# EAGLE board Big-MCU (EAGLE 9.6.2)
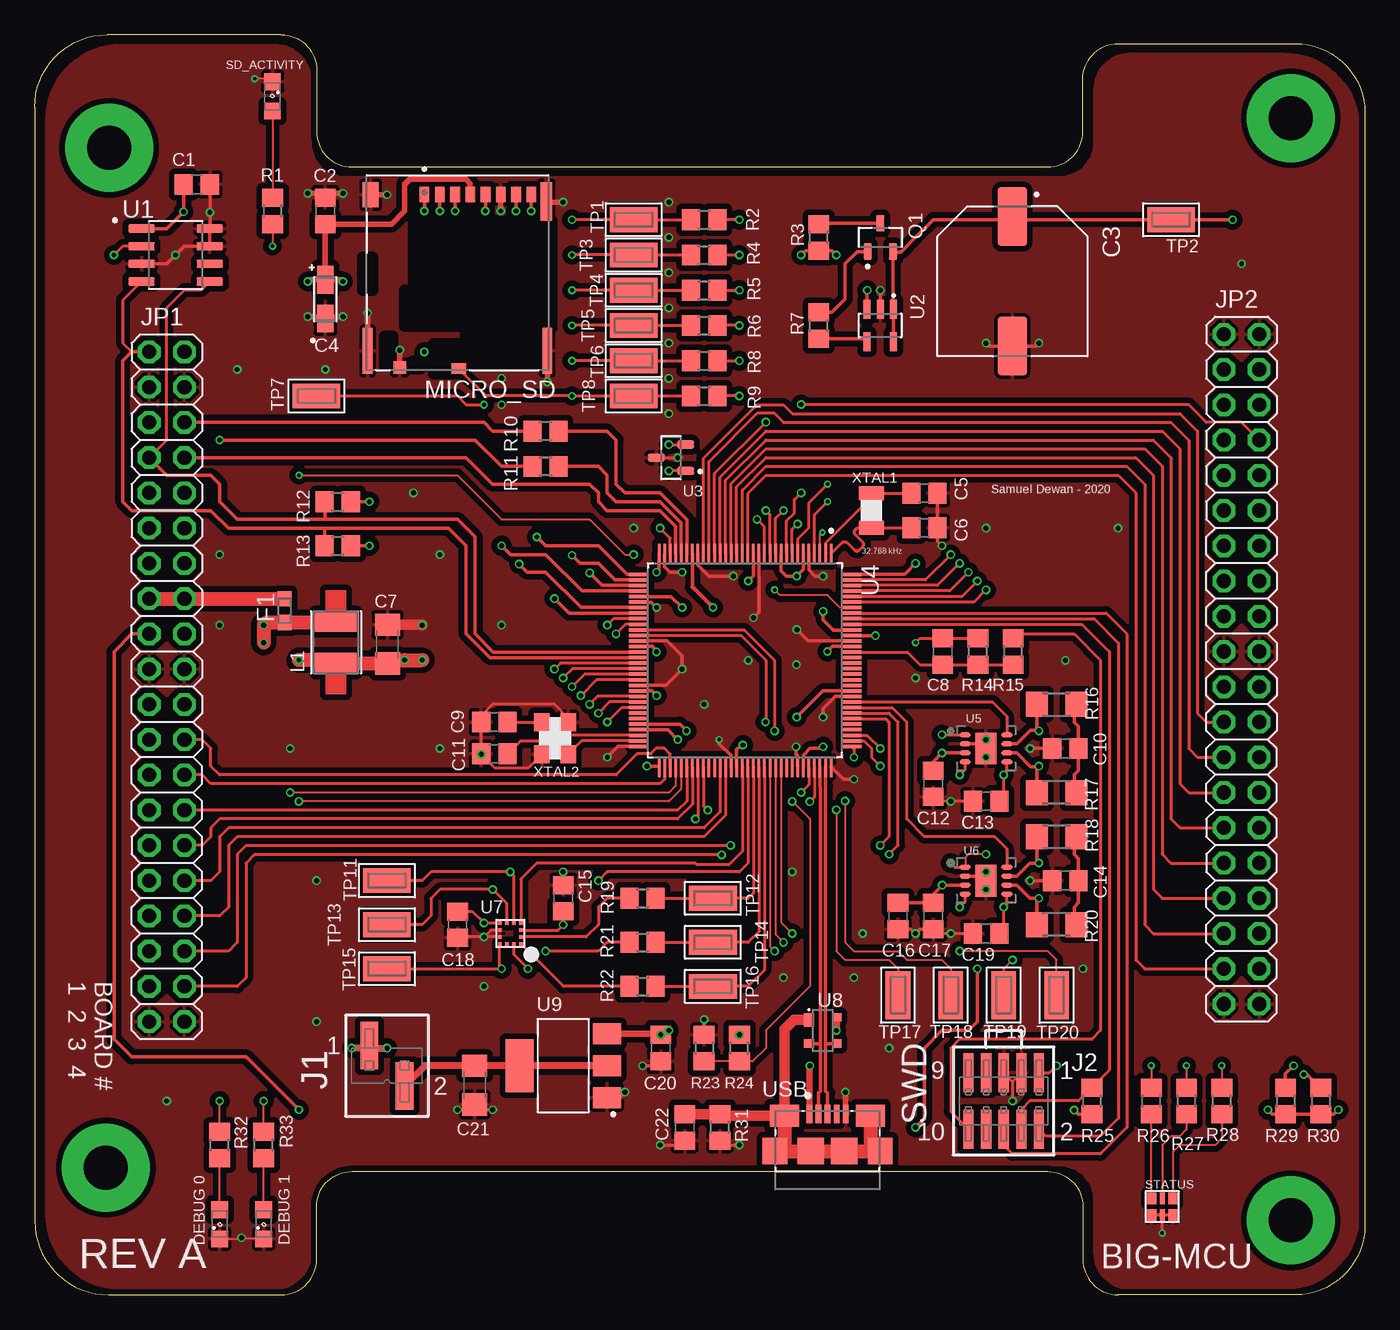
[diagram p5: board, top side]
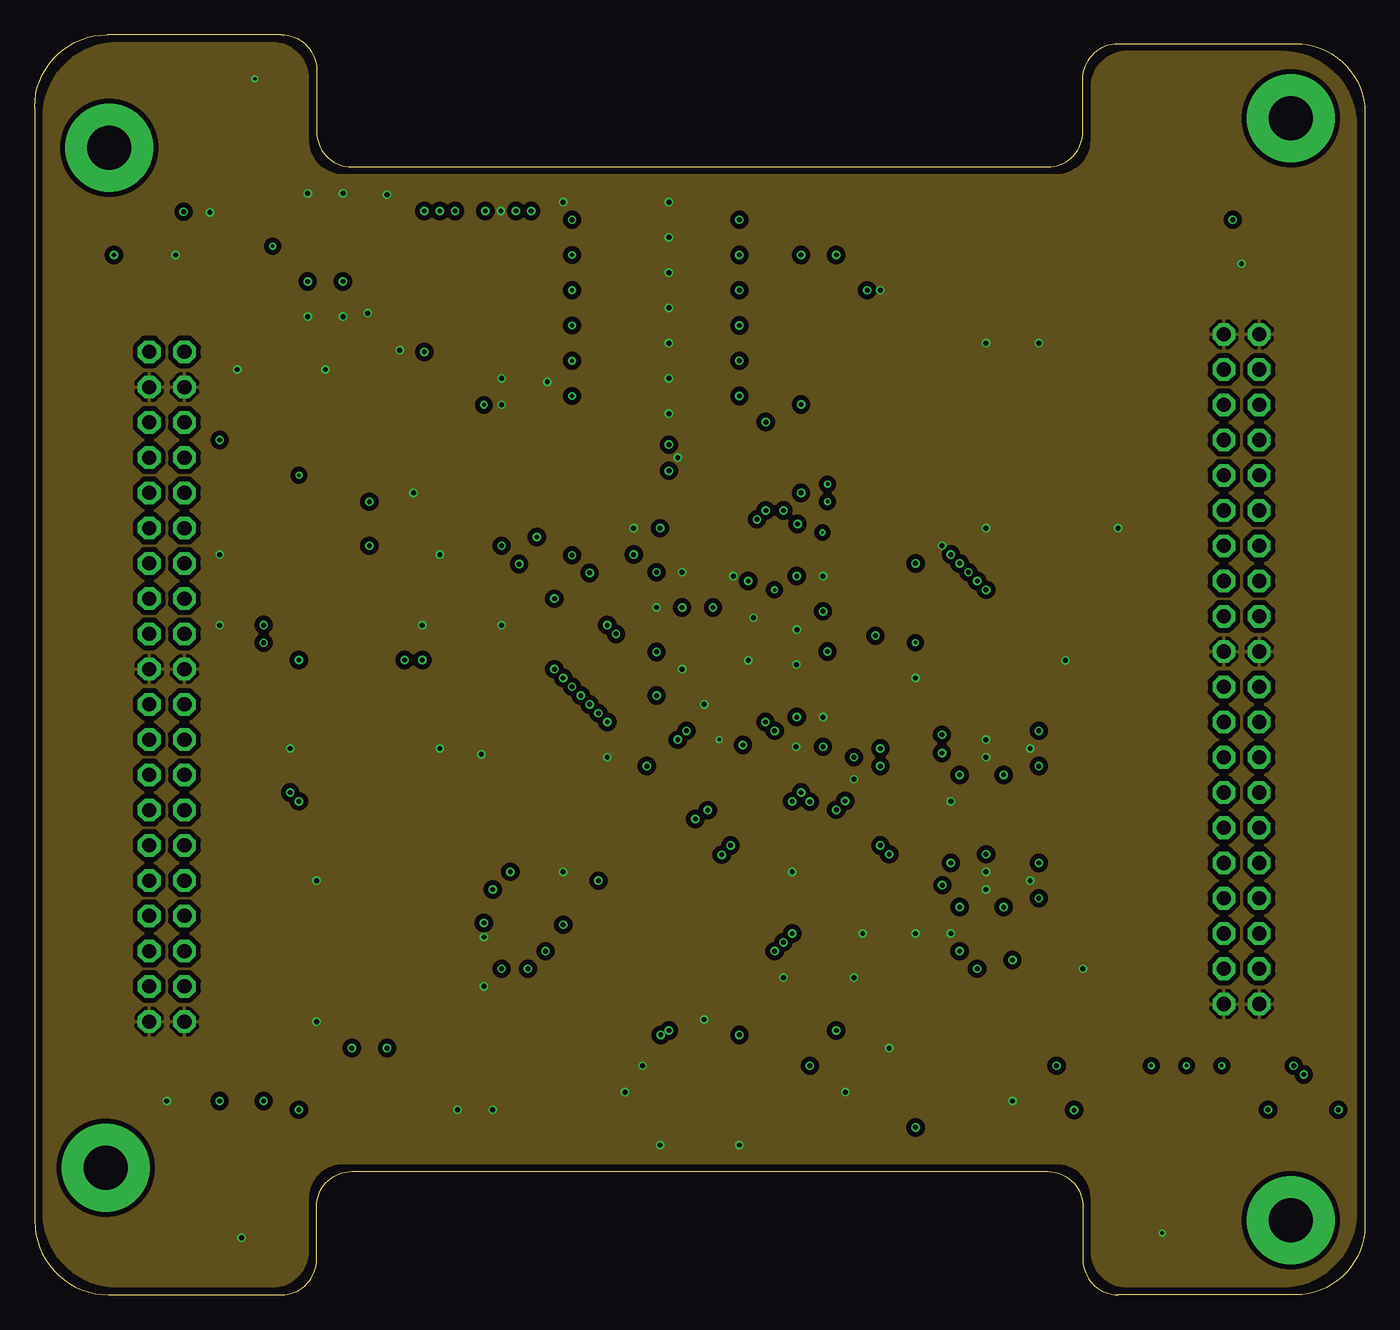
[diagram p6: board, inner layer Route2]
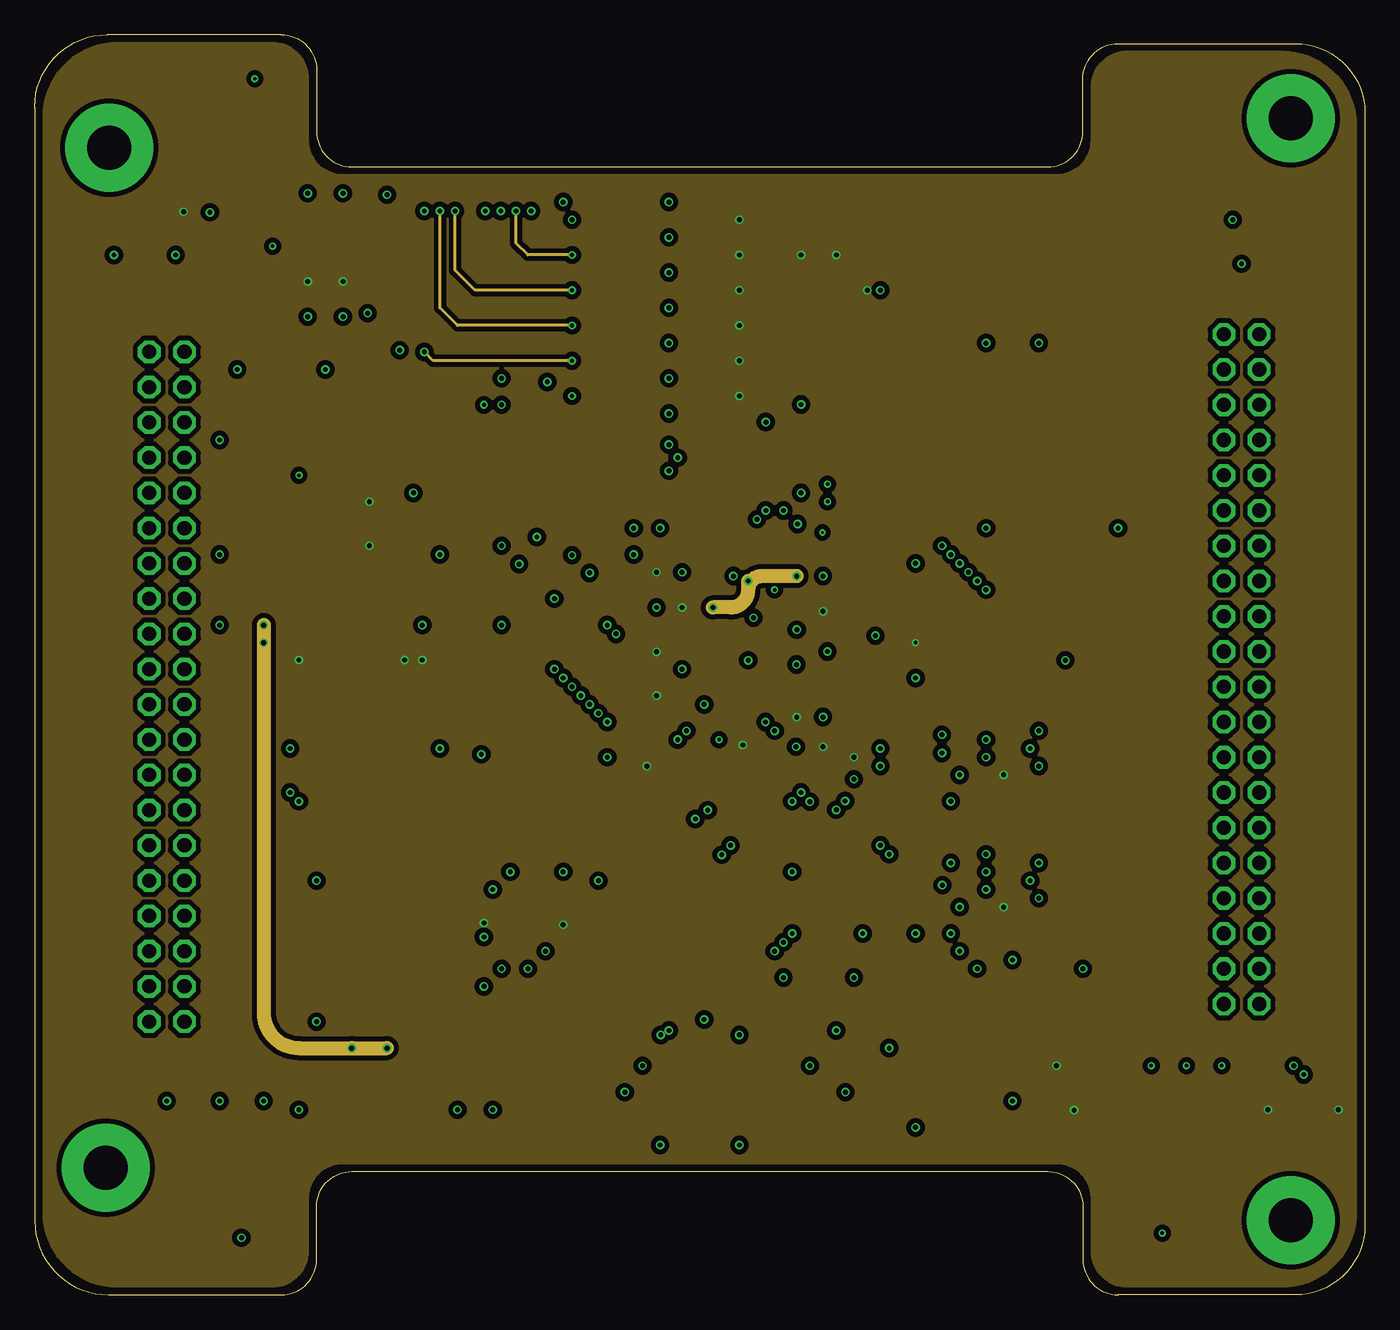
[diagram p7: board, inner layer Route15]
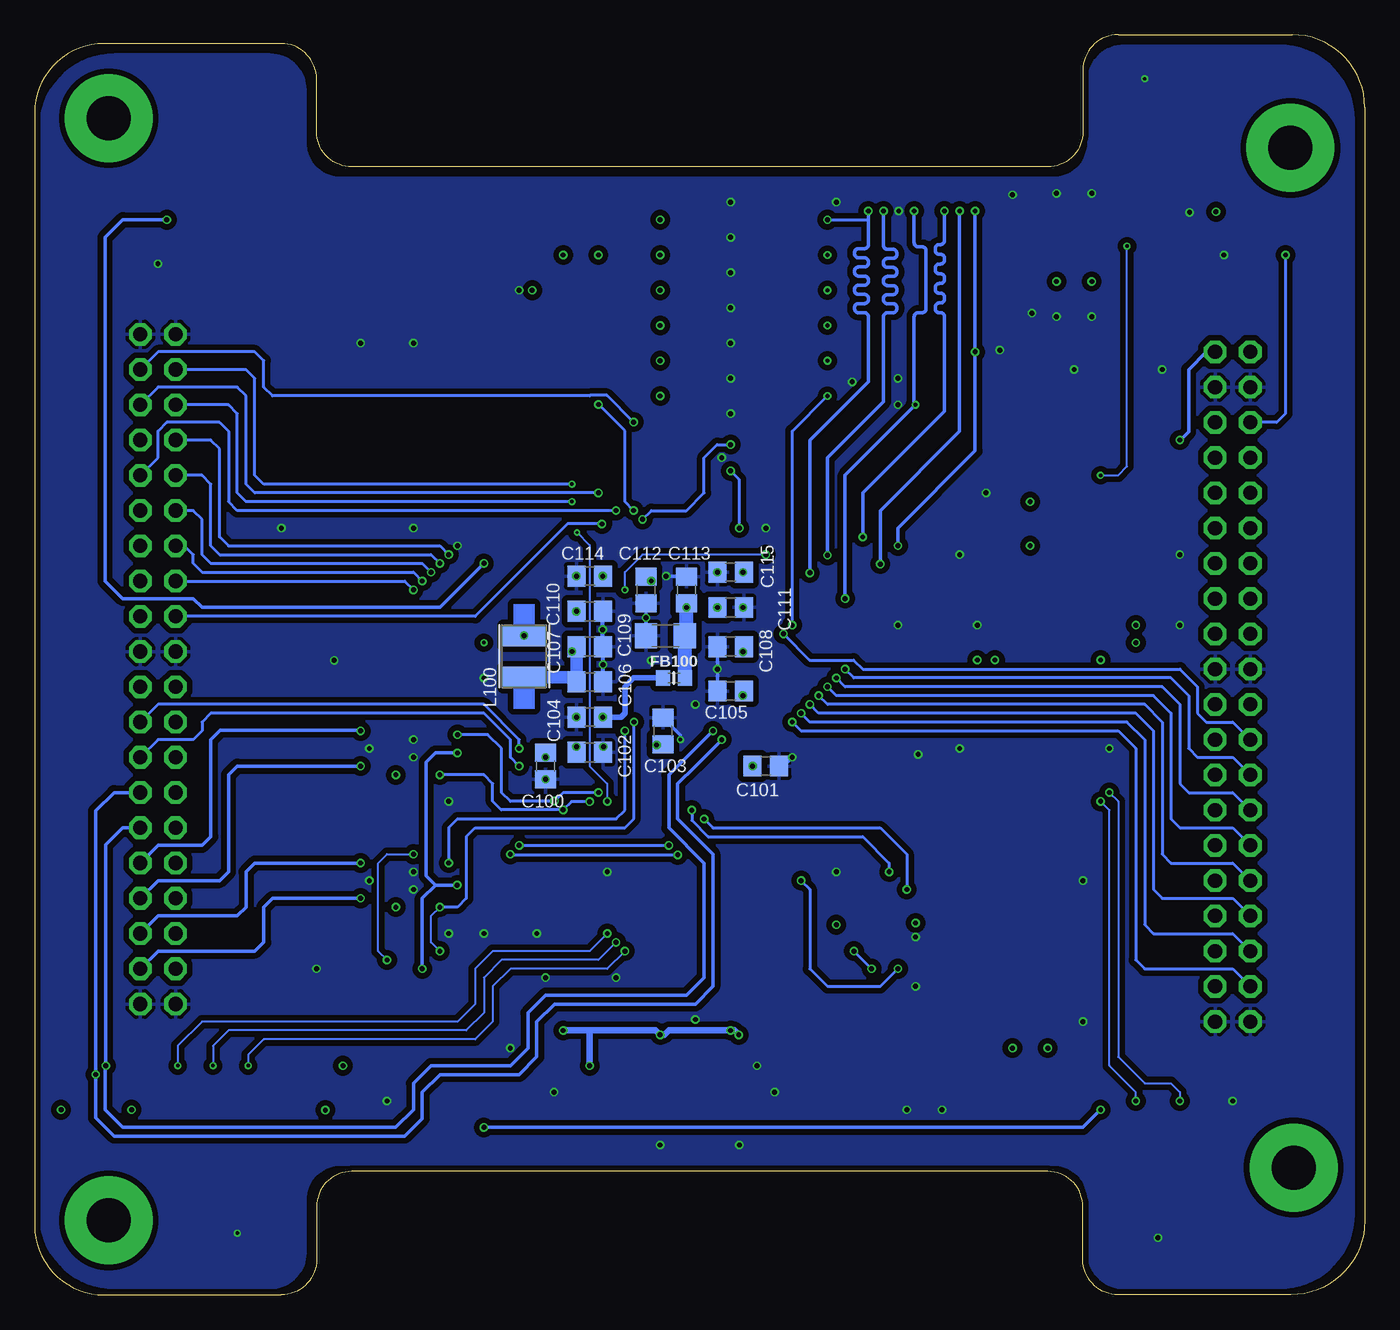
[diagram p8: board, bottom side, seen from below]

Size 95.89 x 90.81 mm. Coordinates in mm from the lower left corner, seen from the top.
Outline: 0,85.57 0,5.33 arc90 5.33,0 17.78,0 arc90 20.32,2.54 20.32,6.35 arc-90 22.86,8.89 73.03,8.89 arc-90 75.56,6.35 75.56,2.54 arc90 78.11,0 90.89,0 arc90 95.89,5 95.89,85.17 arc90 90.89,90.17 78.11,90.17 arc90 75.56,87.63 75.56,83.82 arc-90 73.03,81.28 22.86,81.28 arc-90 20.32,83.82 20.32,88.27 arc90 17.78,90.81 5.23,90.81 arc90 0,85.57
Copper layers (1+2*15+16): Top 0.035mm / dielectric 0.2mm / Route2 0.0175mm / dielectric 1.065mm / Route15 0.0175mm / dielectric 0.2mm / Bottom 0.035mm
Design rules "JLC 4 Layer *": minimum track width 5mil, minimum drill 0.2mm, track to track 3.5mil, track to pad 3.5mil, pad to pad 5mil, via to via 10mil, smd to smd 0mil, copper to edge 10mil, drill to drill 10mil, minimum pad ring 12mil, minimum via ring 5mil, stop-mask expansion 4mil, vias tented up to drill 0mil, thermal gap 10mil
Net classes: 2 diff pairs: width 0.254 mm

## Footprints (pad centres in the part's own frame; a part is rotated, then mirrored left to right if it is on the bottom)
PC/104-MOUNTING-HOLE = drill 3.175 pad 6.35: GND 0,0
C0805 = smd 1.3 x 1.5: 1 -0.95,0; 2 0.95,0
CAPAE1080X580N = smd 4.24 x 2.13: 1 -4.665,0; 2 4.665,0
1206-POL = smd 2 x 1.2: + 1.4,0; - -1.4,0
C1206 = smd 1.6 x 1.8: 1 -1.4,0; 2 1.4,0
SML0805 = smd 1.2 x 1.2: A 1.05,0; C -1.05,0
FUS0603_TYCO = smd 1.092 x 0.991: 1 -0.851,0; 2 0.851,0
0603 = smd 1 x 1.1: 1 -0.794,0; 2 0.794,0
TSM-102-01-L-SV = smd 1.27 x 3.43: 1 -1.27,1.46; 2 1.27,-1.46
SAMTEC-FTSH-105-01-X-DV = smd 0.74 x 2.79: 1 -2.54,-2.032; 2 -2.54,2.032; 3 -1.27,-2.032; 4 -1.27,2.032; 5 0,-2.032; 6 0,2.032; 7 1.27,-2.032; 8 1.27,2.032; 9 2.54,-2.032; 10 2.54,2.032
2X20 = drill 1.016 octagon: 1 -24.13,-1.27; 2 -24.13,1.27; 3 -21.59,-1.27; 4 -21.59,1.27; 5 -19.05,-1.27; 6 -19.05,1.27; 7 -16.51,-1.27; 8 -16.51,1.27; 9 -13.97,-1.27; 10 -13.97,1.27; 11 -11.43,-1.27; 12 -11.43,1.27; 13 -8.89,-1.27; 14 -8.89,1.27; 15 -6.35,-1.27; 16 -6.35,1.27; 17 -3.81,-1.27; 18 -3.81,1.27; 19 -1.27,-1.27; 20 -1.27,1.27; 21 1.27,-1.27; 22 1.27,1.27; 23 3.81,-1.27; 24 3.81,1.27; 25 6.35,-1.27; 26 6.35,1.27; 27 8.89,-1.27; 28 8.89,1.27; 29 11.43,-1.27; 30 11.43,1.27; 31 13.97,-1.27; 32 13.97,1.27; 33 16.51,-1.27; 34 16.51,1.27; 35 19.05,-1.27; 36 19.05,1.27; 37 21.59,-1.27; 38 21.59,1.27; 39 24.13,-1.27; 40 24.13,1.27
LQH43PN100M26L = smd 1.5 x 3: 1 -1.5,0; 2 1.5,0
MOLEX_503398-1892 = smd 0.7 x 1.1: 1 -3.65,6.895; 2 -2.55,6.895; 3 -1.45,6.895; 4 -0.35,6.895; 5 0.75,6.895; 6 1.85,6.895; 7 2.95,6.895; 8 4.05,6.895 | smd 0.9 x 0.93: 9 -5.44,-5.57 | smd 1.05 x 0.78: 10 -1.175,-5.645 | smd 1.14 x 1.83: P1 -7.53,6.88 | smd 0.86 x 2.8: P2 5.13,6.395 | smd 0.7 x 3.33: P3 -7.75,-4.37; P4 5.21,-4.37
SOT91P240X110-3N = smd 1.18 x 0.61: 1 -1.025,0.915; 2 -1.025,-0.915; 3 1.025,0
R0805 = smd 1.3 x 1.5: 1 -0.95,0; 2 0.95,0
R1206 = smd 1.6 x 1.803: 1 -1.422,0; 2 1.422,0
MSL0402RGB = smd 0.67 x 0.83: P1 0.77,-0.585; P3 -0.77,-0.585; P4 0.77,0.585; P6 -0.77,0.585 | smd 0.37 x 0.83: P2 0,-0.585; P5 0,0.585
KEYSTONE_5015 = smd 3.43 x 1.78: 1 0,0
SOIC8 = smd 1.91 x 0.6: 1 -2.46,1.905; 2 -2.46,0.635; 3 -2.46,-0.635; 4 -2.46,-1.905; 5 2.46,-1.905; 6 2.46,-0.635; 7 2.46,0.635; 8 2.46,1.905
SOT95P285X145-5N = smd 1.37 x 0.59: 1 -1.175,0.95; 2 -1.175,0; 3 -1.175,-0.95; 4 1.175,-0.95; 5 1.175,0.95
SOT95P237X112-3N = smd 1.23 x 0.59: 1 -1.06,0.95; 2 -1.06,-0.95; 3 1.06,0
QFP40P1600X1600X120-128N = smd 1.47 x 0.24: 1 -7.67,6.2; 2 -7.67,5.8; 3 -7.67,5.4; 4 -7.67,5; 5 -7.67,4.6; 6 -7.67,4.2; 7 -7.67,3.8; 8 -7.67,3.4; 9 -7.67,3; 10 -7.67,2.6; 11 -7.67,2.2; 12 -7.67,1.8; 13 -7.67,1.4; 14 -7.67,1; 15 -7.67,0.6; 16 -7.67,0.2; 17 -7.67,-0.2; 18 -7.67,-0.6; 19 -7.67,-1; 20 -7.67,-1.4; 21 -7.67,-1.8; 22 -7.67,-2.2; 23 -7.67,-2.6; 24 -7.67,-3; 25 -7.67,-3.4; 26 -7.67,-3.8; 27 -7.67,-4.2; 28 -7.67,-4.6; 29 -7.67,-5; 30 -7.67,-5.4; 31 -7.67,-5.8; 32 -7.67,-6.2; 65 7.67,-6.2; 66 7.67,-5.8; 67 7.67,-5.4; 68 7.67,-5; 69 7.67,-4.6; 70 7.67,-4.2; 71 7.67,-3.8; 72 7.67,-3.4; 73 7.67,-3; 74 7.67,-2.6; 75 7.67,-2.2; 76 7.67,-1.8; 77 7.67,-1.4; 78 7.67,-1; 79 7.67,-0.6; 80 7.67,-0.2; 81 7.67,0.2; 82 7.67,0.6; 83 7.67,1; 84 7.67,1.4; 85 7.67,1.8; 86 7.67,2.2; 87 7.67,2.6; 88 7.67,3; 89 7.67,3.4; 90 7.67,3.8; 91 7.67,4.2; 92 7.67,4.6; 93 7.67,5; 94 7.67,5.4; 95 7.67,5.8; 96 7.67,6.2 | smd 0.24 x 1.47: 33 -6.2,-7.67; 34 -5.8,-7.67; 35 -5.4,-7.67; 36 -5,-7.67; 37 -4.6,-7.67; 38 -4.2,-7.67; 39 -3.8,-7.67; 40 -3.4,-7.67; 41 -3,-7.67; 42 -2.6,-7.67; 43 -2.2,-7.67; 44 -1.8,-7.67; 45 -1.4,-7.67; 46 -1,-7.67; 47 -0.6,-7.67; 48 -0.2,-7.67; 49 0.2,-7.67; 50 0.6,-7.67; 51 1,-7.67; 52 1.4,-7.67; 53 1.8,-7.67; 54 2.2,-7.67; 55 2.6,-7.67; 56 3,-7.67; 57 3.4,-7.67; 58 3.8,-7.67; 59 4.2,-7.67; 60 4.6,-7.67; 61 5,-7.67; 62 5.4,-7.67; 63 5.8,-7.67; 64 6.2,-7.67; 97 6.2,7.67; 98 5.8,7.67; 99 5.4,7.67; 100 5,7.67; 101 4.6,7.67; 102 4.2,7.67; 103 3.8,7.67; 104 3.4,7.67; 105 3,7.67; 106 2.6,7.67; 107 2.2,7.67; 108 1.8,7.67; 109 1.4,7.67; 110 1,7.67; 111 0.6,7.67; 112 0.2,7.67; 113 -0.2,7.67; 114 -0.6,7.67; 115 -1,7.67; 116 -1.4,7.67; 117 -1.8,7.67; 118 -2.2,7.67; 119 -2.6,7.67; 120 -3,7.67; 121 -3.4,7.67; 122 -3.8,7.67; 123 -4.2,7.67; 124 -4.6,7.67; 125 -5,7.67; 126 -5.4,7.67; 127 -5.8,7.67; 128 -6.2,7.67
VDFN8 = smd 2.3 x 1.5: EP 0,0 | smd 0.35 x 0.8: P1 -0.975,-1.5; P2 -0.325,-1.5; P3 0.325,-1.5; P4 0.975,-1.5; P5 0.975,1.5; P6 0.325,1.5; P7 -0.325,1.5; P8 -0.975,1.5
KX134-1211 = smd 0.275 x 0.25: 1 -0.762,0.75; 2 -0.762,0.25; 3 -0.762,-0.25; 4 -0.762,-0.75; 7 0.762,-0.75; 8 0.762,-0.25; 9 0.762,0.25; 10 0.762,0.75 | smd 0.25 x 0.275: 5 -0.25,-0.762; 6 0.25,-0.762; 11 0.25,0.762; 12 -0.25,0.762
SOT143B = smd 1 x 0.7: 1 -0.75,-1 | smd 0.6 x 0.7: 2 0.95,-1; 3 0.95,1; 4 -0.95,1
SOT223 = smd 1.5 x 2: 1 -2.3,-3.15; 2 0,-3.15; 3 2.3,-3.15 | smd 3.8 x 2: 4 0,3.15
10118192-0001LF = smd 0.4 x 1.35: 1 -1.3,2.54; 2 -0.65,2.54; 3 0,2.54; 4 0.65,2.54; 5 1.3,2.54 | smd 2.1 x 1.6: SH1 -3.1,2.415; SH2 3.1,2.415 | smd 1.8 x 1.9: SH3 -3.8,-0.135; SH6 3.8,-0.135 | smd 1.9 x 1.9: SH4 -1.2,-0.135; SH5 1.2,-0.135
CM7V-T1A-32.768KHZ-12.5PF-10PPM-TA-QC = smd 1 x 1.8: P$1 -1.25,0; P$2 1.25,0
RH100-12.000-12-1010-EXT-TR = smd 1.3 x 1.1: P1 -1.15,-0.95; P2 1.15,-0.95; P3 1.15,0.95; P4 -1.15,0.95

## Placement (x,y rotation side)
$$U$1  PS/104-MOUNTING-HOLE  [PC/104-MOUNTING-HOLE]  5.13,9.17 0 top
C1  0.1 µF  [C0805]  11.68,80.01 0 top
C2  0.1 µF  [C0805]  20.95,78.11 90 top
C3  FC0H473ZFTBR24  [CAPAE1080X580N]  70.48,73.03 270 top
C4  TAJA106K010RNJ  [1206-POL]  20.95,71.75 90 top
C5  22 pF  [C0805]  64.14,57.76 180 top
C6  22 pF  [C0805]  64.14,55.27 180 top
C7  10 µF  [C1206]  25.43,46.89 90 top
C8  100 pF  [C0805]  65.46,46.35 270 top
C9  18 pF  [C0805]  33.15,41.27 0 top
C10  4.7 µF  [C0805]  74.3,39.37 180 top
C11  18 pF  [C0805]  33.15,38.99 0 top
C12  0.1 µF  [C0805]  64.77,36.83 90 top
C13  0.1 µF  [C0805]  68.58,35.56 0 top
C14  4700 pF  [C0805]  74.3,29.84 180 top
C15  0.1µF  [C0805]  38.1,28.57 90 top
C16  4.7 µF  [C0805]  62.23,27.3 90 top
C17  0.1 µF  [C0805]  64.77,27.3 90 top
C18  0.1 µF  [C0805]  30.48,26.67 270 top
C19  0.1 µF  [C0805]  68.58,26.04 0 top
C20  0.1 µF  [C0805]  45.14,17.78 270 top
C21  10 µF  [C1206]  31.72,15.11 270 top
C22  4.7 nF  [C0805]  46.86,12.06 270 top
C100  0.1 µF  [C0805]  59.05,38.1 270 bottom
C101  0.1 µF  [C0805]  43.18,38.1 0 bottom
C102  0.1 µF  [C0805]  55.88,39.09 0 bottom
C103  0.1 µF  [C0805]  50.6,40.64 90 bottom
C104  0.1 µF  [C0805]  55.88,41.63 180 bottom
C105  0.1 µF  [C0805]  45.72,43.51 180 bottom
C106  4.7 µF  [C0805]  55.88,44.17 0 bottom
C107  0.1 µF  [C0805]  55.88,46.71 0 bottom
C108  0.1 µF  [C0805]  45.72,46.71 180 bottom
C109  10 µF  [C1206]  50.42,47.5 180 bottom
C110  0.1 µF  [C0805]  55.88,49.25 0 bottom
C111  0.1 µF  [C0805]  45.72,49.53 0 bottom
C112  0.1 µF  [C0805]  51.82,50.8 270 bottom
C113  0.1 µF  [C0805]  48.9,50.8 90 bottom
C114  0.1 µF  [C0805]  55.88,51.79 180 bottom
C115  0.1 µF  [C0805]  45.72,52.07 180 bottom
DEBUG1  [SML0805]  13.34,5.08 90 top
DEBUG2  [SML0805]  16.51,5.08 90 top
F1  0603SFF150F/32-2  [FUS0603_TYCO]  18.02,49.3 270 top
FB100  BLM18PG471SN1D  [0603]  49.81,44.45 0 bottom
J1  TSM-102-01-L-SVJ  [TSM-102-01-L-SV]  25.4,16.51 0 top
J2  SAMTEC-FTSH-105-01-X-DVJ  [SAMTEC-FTSH-105-01-X-DV]  69.85,13.97 180 top
JP1  [2X20]  9.53,43.81 270 top
JP2  [2X20]  87,45.09 270 top
L1  LQH43PN100M26L  [LQH43PN100M26L]  21.72,47.02 270 top
L100  LQH43PN100M26L  [LQH43PN100M26L]  60.6,46 270 bottom
MICRO_SD  503398-1892  [MOLEX_503398-1892]  31.75,72.39 0 top
Q1  DMG2305UX-13  [SOT91P240X110-3N]  60.96,76.2 90 top
R1  22 kΩ  [R0805]  17.14,78.11 270 top
R2  100 kΩ  [R0805]  48.26,77.47 0 top
R3  220 Ω  [R0805]  56.52,76.2 90 top
R4  100 kΩ  [R0805]  48.26,74.93 0 top
R5  10 kΩ  [R0805]  48.26,72.39 0 top
R6  100 kΩ  [R0805]  48.26,69.85 0 top
R7  1 kΩ  [R0805]  56.52,69.85 90 top
R8  100 kΩ  [R0805]  48.26,67.31 0 top
R9  10 kΩ  [R0805]  48.26,64.77 0 top
R10  33 Ω  [R0805]  36.83,62.23 180 top
R11  33 Ω  [R0805]  36.83,59.69 180 top
R12  2.2 kΩ  [R0805]  21.84,57.15 0 top
R13  2.2 kΩ  [R0805]  21.84,53.98 0 top
R14  2.2 kΩ  [R0805]  68,46.35 90 top
R15  330 Ω  [R0805]  70.54,46.35 90 top
R16  60.4 Ω  [R1206]  73.66,42.55 180 top
R17  60.4 Ω  [R1206]  73.66,36.2 0 top
R18  60.4 Ω  [R1206]  73.66,33.02 180 top
R19  33 Ω  [R0805]  43.81,28.57 0 top
R20  60.4 Ω  [R1206]  73.66,26.67 0 top
R21  33 Ω  [R0805]  43.81,25.4 0 top
R22  33 Ω  [R0805]  43.81,22.23 0 top
R23  10 kΩ  [R0805]  48.26,17.78 270 top
R24  91 kΩ  [R0805]  50.8,17.78 90 top
R25  1 kΩ  [R0805]  76.2,13.97 270 top
R26  330 Ω  [R0805]  80.49,13.97 90 top
R27  330 Ω  [R0805]  83.03,13.97 90 top
R28  330 Ω  [R0805]  85.57,13.97 90 top
R29  2.2 kΩ  [R0805]  90.17,13.97 270 top
R30  2.2 kΩ  [R0805]  92.71,13.97 270 top
R31  1 MΩ  [R0805]  49.4,12.06 90 top
R32  22 kΩ  [R0805]  13.34,10.79 90 top
R33  22 kΩ  [R0805]  16.51,10.79 90 top
SD_ACTIVITY  [SML0805]  17.14,86.36 270 top
STATUS  MSL0402RGB  [MSL0402RGB]  81.28,6.35 0 top
TP1  5015  [KEYSTONE_5015]  43.18,77.47 0 top
TP2  5015  [KEYSTONE_5015]  81.92,77.47 180 top
TP3  5015  [KEYSTONE_5015]  43.18,74.93 0 top
TP4  5015  [KEYSTONE_5015]  43.18,72.39 0 top
TP5  5015  [KEYSTONE_5015]  43.18,69.85 0 top
TP6  5015  [KEYSTONE_5015]  43.18,67.31 0 top
TP7  5015  [KEYSTONE_5015]  20.32,64.77 0 top
TP8  5015  [KEYSTONE_5015]  43.18,64.77 0 top
TP11  5015  [KEYSTONE_5015]  25.4,29.84 0 top
TP12  5015  [KEYSTONE_5015]  48.9,28.57 0 top
TP13  5015  [KEYSTONE_5015]  25.4,26.67 0 top
TP14  5015  [KEYSTONE_5015]  48.9,25.4 0 top
TP15  5015  [KEYSTONE_5015]  25.4,23.5 0 top
TP16  5015  [KEYSTONE_5015]  48.9,22.23 0 top
TP17  5015  [KEYSTONE_5015]  62.23,21.59 270 top
TP18  5015  [KEYSTONE_5015]  66.04,21.59 270 top
TP19  5015  [KEYSTONE_5015]  69.85,21.59 270 top
TP20  5015  [KEYSTONE_5015]  73.66,21.59 270 top
U1  DS2482-100  [SOIC8]  10.16,74.93 0 top
U2  BU7265SG-TR  [SOT95P285X145-5N]  60.96,69.85 270 top
U3  TC1046VNBTR  [SOT95P237X112-3N]  45.87,60.33 180 top
U4  ATSAMD51P20A-AU  [QFP40P1600X1600X120-128N]  51.21,45.72 270 top
U5  ATA6561  [VDFN8]  68.58,39.37 270 top
U6  ATA6561  [VDFN8]  68.58,29.84 270 top
U7  [KX134-1211]  34.29,26.04 180 top
U8  PRTR5V0U2X_215  [SOT143B]  56.82,19.05 270 top
U9  LDL1117S33R  [SOT223]  38.1,16.51 90 top
U$1  PS/104-MOUNTING-HOLE  [PC/104-MOUNTING-HOLE]  90.55,84.79 0 top
U$2  PS/104-MOUNTING-HOLE  [PC/104-MOUNTING-HOLE]  5.36,82.65 0 top
U$3  PS/104-MOUNTING-HOLE  [PC/104-MOUNTING-HOLE]  90.55,5.36 0 top
USB  10118192-0001LF  [10118192-0001LF]  57.15,10.49 0 top
XTAL1  CM7V-T1A  [CM7V-T1A-32.768KHZ-12.5PF-10PPM-TA-QC]  60.33,56.52 90 top
XTAL2  RH100-12.000-12-1010-EXT-TR  [RH100-12.000-12-1010-EXT-TR]  37.52,40.11 90 top

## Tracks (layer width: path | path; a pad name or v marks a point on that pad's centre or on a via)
1W  (via drill 0.35)
  Top 0.203: U1.2 6.35,75.56 v5.71,74.93
  Bottom 0.203: v5.71,74.93 5.71,63.5 6.35,62.87 JP1.5
3.3V  (via drill 0.35)
  Top 0.508: v22.86,17.78 23.94,17.78 J1.1 24.32,17.78 v25.4,17.78
  Top 1.016: L1.1 21.65,48.45 F1.2 16.7,48.45 v16.51,48.26 v16.51,46.99
  Route15 1.016: v16.51,48.26 v16.51,46.99 16.51,20.32 arc90 19.05,17.78 v22.86,17.78 v25.4,17.78
+5V  (via drill 0.35)
  Top 0.203: 64.77,28.57 C17.2
  Top 0.254: v63.5,12.06 64.14,12.7 64.14,17.78 65.41,19.05 67.31,19.05 67.94,19.68 v67.94,23.5 | v19.05,13.34 15.24,17.14 6.99,17.14 5.71,18.41 5.71,46.35 6.99,47.62 JP1.17 | C16.2 64.45,28.25 64.77,28.57 | U5.P3 v65.41,39.05 64.77,38.41 C12.2 | C17.2 64.77,28.86 v65.43,29.52 U6.P3
  Bottom 0.254: v65.41,39.05 67,39.05 67.67,38.38 67.67,30.19 67,29.52 | v19.05,13.34 20.32,12.06 v63.5,12.06 | v65.43,29.52 67,29.52 | 67,29.52 67.94,28.57 v67.94,23.5
A0  (via drill 0.25)
  Top 0.203: U4.7 55.01,54.47 55.8,55.27 55.8,57.07 v57.15,58.42
  Bottom 0.203: JP2.3 80.64,66.67 80.01,66.04 80.01,59.05 79.38,58.42 v57.15,58.42
A1  (via drill 0.25)
  Top 0.203: U4.4 56.21,56.21 v57.15,57.15
  Bottom 0.203: JP2.5 81.92,64.14 81.28,63.5 81.28,57.78 80.64,57.15 v57.15,57.15
A2  (via drill 0.35)
  Top 0.203: U4.127 64.22,51.52 v66.04,53.34
  Bottom 0.203: JP2.7 83.19,61.59 82.55,60.96 82.55,54.61 81.92,53.98 66.67,53.98 v66.04,53.34
A3  (via drill 0.35)
  Top 0.203: U4.126 65.09,51.12 v66.67,52.7
  Bottom 0.203: JP2.9 83.82,59.05 83.19,58.42 83.19,53.98 82.55,53.34 67.31,53.34 v66.67,52.7
A4  (via drill 0.35)
  Top 0.203: U4.125 65.96,50.72 v67.31,52.07
  Bottom 0.203: JP2.11 84.45,56.52 83.82,55.88 83.82,53.34 83.19,52.7 67.94,52.7 v67.31,52.07
A5  (via drill 0.35)
  Top 0.203: U4.124 66.83,50.32 v67.94,51.44
  Bottom 0.203: JP2.13 85.09,53.98 84.45,53.34 84.45,52.7 83.82,52.07 68.58,52.07 v67.94,51.44
A6  (via drill 0.35)
  Top 0.203: U4.123 67.7,49.92 v68.58,50.8
  Bottom 0.203: JP2.15 69.22,51.44 v68.58,50.8
A7  (via drill 0.35)
  Top 0.203: U4.8 54.61,55.16 v54.99,55.55
  Bottom 0.203: JP2.17 64.14,48.9 57.48,55.55 v54.99,55.55
A12  (via drill 0.35)
  Top 0.203: U4.11 53.41,55.95 v53.98,56.52
  Bottom 0.203: v53.98,56.52 81.28,56.52 81.92,57.15 81.92,62.23 82.55,62.87 86.36,62.87 87,62.23 87,60.33 JP2.10
A13  (via drill 0.35)
  Top 0.203: U4.12 53.01,56.21 v52.7,56.52 | v55.24,64.16 83.16,64.16 84.45,62.87 87,62.87 JP2.8
  Bottom 0.203: v52.7,56.52 53.34,57.15 53.34,62.25 v55.24,64.16
ACCEL_CS  (via drill 0.35)
  Top 0.203: U4.81 51.41,31.09 50.8,30.48 41.27,30.48 v40.64,29.84 | U7.10 33.53,23.62 v33.66,23.5 TP15.1
  Bottom 0.203: v40.64,29.84 40.01,29.21 40.01,23.5 38.73,22.23 34.92,22.23 v33.66,23.5
ACCEL_INT_1  (via drill 0.35)
  Top 0.203: U4.73 48.21,35.23 v48.51,34.92 | U7.5 34.54,30.23 v34.29,30.48 28.57,30.48 27.94,29.84 TP11.1
  Bottom 0.203: v48.51,34.92 48.51,34.19 47.35,33.02 36.2,33.02 34.29,31.11 v34.29,30.48
ACCEL_INT_2  (via drill 0.35)
  Top 0.203: U4.72 47.81,34.47 v47.62,34.29 | U7.6 34.04,28.19 v33.02,29.21 29.21,29.21 28.57,28.57 28.57,27.3 27.94,26.67 TP13.1
  Bottom 0.203: v47.62,34.29 46.99,33.66 34.92,33.66 33.02,31.75 v33.02,29.21
ACCEL_TRIG
  Top 0.203: U4.80 51.01,31.96 50.04,30.99 47.75,30.99 47.62,31.11 36.2,31.11 35.05,29.97 U7.4
CAN0_H  (via drill 0.35)
  Top 0.254: U5.P7 70.81,39.7 71.79,40.68 72.35,40.68 v72.39,40.64 72.24,40.79 R16.2
  Bottom 0.254: JP2.32 87,32.38 83.82,32.38 83.19,33.02 83.19,40.01 82.51,40.68 72.43,40.68 v72.39,40.64
CAN0_L  (via drill 0.35)
  Top 0.254: U5.P6 70.81,39.05 71.79,38.06 72.35,38.06 v72.39,38.1 72.24,37.95 R17.1
  Bottom 0.254: JP2.34 87,29.84 82.55,29.84 81.92,30.48 81.92,37.47 81.28,38.1 v72.39,38.1
CAN0_RX  (via drill 0.35)
  Top 0.152: TP17.1 62.23,23.5 61.59,24.13 58.42,24.13 57.78,24.77 v57.78,34.95
  Top 0.203: U4.93 56.21,35.86 v55.88,35.54 | v66.67,37.47 67.08,37.87 U5.P4
  Bottom 0.203: v66.67,37.47 63.5,37.47 62.87,36.83 62.87,35.56 62.25,34.95 v57.78,34.95 57.2,35.54 v55.88,35.54
CAN0_STBY
  Top 0.203: U5.P8 70.08,41.68 69.04,42.72 U4.105
CAN0_TX  (via drill 0.35)
  Top 0.152: TP18.1 66.04,23.5 65.41,24.13 62.87,24.13 62.23,24.77 59.05,24.77 58.42,25.4 v58.42,35.58
  Top 0.203: U4.92 55.81,36.76 v55.24,36.2 | v65.41,40.36 67.06,40.36 U5.P1
  Bottom 0.203: 58.42,35.56 57.78,36.2 v55.24,36.2 | v58.42,35.58 58.42,35.56 | 58.42,35.56 61.59,35.56 62.23,36.2 62.23,39.37 63.22,40.36 v65.41,40.36
CAN1_H  (via drill 0.35)
  Top 0.254: U6.P7 70.81,30.17 71.75,31.11 v72.39,31.11 72.24,31.27 R18.2
  Bottom 0.254: JP2.36 87,27.3 81.28,27.3 80.64,27.94 80.64,30.48 80.01,31.11 v72.39,31.11
CAN1_L  (via drill 0.35)
  Top 0.254: U6.P6 70.81,29.52 71.75,28.57 v72.39,28.57 72.24,28.42 R20.1
  Bottom 0.254: JP2.38 87,24.77 80.01,24.77 79.38,25.4 79.38,27.94 78.74,28.57 v72.39,28.57
CAN1_RX  (via drill 0.35)
  Top 0.152: TP20.1 73.66,24.13 73.03,24.77 v66.67,24.77
  Top 0.203: U4.44 50.91,47.52 52.7,45.72 52.7,41.3 v52.68,41.27 | v66.67,27.94 67.08,28.34 U6.P4
  Bottom 0.152: v66.67,24.77 67.31,25.4 67.31,27.3 v66.67,27.94
  Bottom 0.203: v52.68,41.27 52.68,34.31 53.34,33.66 64.14,33.66 64.77,33.02 64.77,28.57 65.41,27.94 v66.67,27.94
CAN1_STBY
  Top 0.203: U4.104 61.82,42.32 62.87,41.27 62.87,34.29 64.14,33.02 69.22,33.02 70.08,32.16 U6.P8
CAN1_TX  (via drill 0.35)
  Top 0.152: TP19.1 69.85,23.5 v70.48,24.13 | U6.P1 67.08,31.52 67.31,31.75 v68.58,31.75
  Top 0.203: U4.43 51.14,47.92 53.34,45.72 v53.34,40.64 | v66.04,31.11 66.33,30.82 U6.P1
  Bottom 0.152: v70.48,24.13 71.12,24.77 71.12,31.11 70.48,31.75 v68.58,31.75
  Bottom 0.203: v53.34,40.64 53.34,34.92 53.98,34.29 65.41,34.29 66.04,33.66 v66.04,31.11
DAC0  (via drill 0.35)
  Top 0.203: U4.22 49.01,59.19 v52.7,62.89
  Bottom 0.203: JP2.4 87,67.94 80.01,67.94 79.38,67.31 79.38,65.41 78.74,64.77 55.88,64.77 55.84,64.81 54.63,64.81 v52.7,62.89
DAC1  (via drill 0.35)
  Top 0.203: U4.9 54.21,55.78 54.76,56.34 54.76,57.3 v55.24,57.78
  Bottom 0.203: JP2.6 87,65.41 81.28,65.41 80.64,64.77 80.64,58.42 80.01,57.78 v55.24,57.78
DEBUG_0  (via drill 0.35)
  Top 0.152: U4.68 46.21,36.68 45.72,36.2 v18.41,36.2 | R32.2 v13.34,13.97
  Bottom 0.152: v18.41,36.2 17.78,35.56 17.78,17.14 15.88,15.24 13.97,15.24 13.34,14.61 v13.34,13.97
DEBUG_1  (via drill 0.35)
  Top 0.152: U4.69 46.61,36.45 45.72,35.56 v19.05,35.56 | R33.2 v16.51,13.97
  Bottom 0.152: v19.05,35.56 18.41,34.92 18.41,16.51 16.51,14.61 v16.51,13.97
GND  (via drill 0.25, 0.35)
  Top 0.152: SD_ACTIVITY.C 16.93,87.63 v15.88,87.63 | C15.2 v38.1,30.48 | DEBUG2.C 14.99,4.03 v14.91,4.12 14.82,4.03 DEBUG1.C
  Top 0.203: STATUS.P3 STATUS.P2 | STATUS.P2 STATUS.P1 | DEBUG1.C 13.55,3.76 | U3.3 v46.35,60.33 | C6.1 65.08,55.56 | 65.08,57.47 C5.1 | XTAL2.P4 35.56,37.95 33.2,37.95 v32.2,38.95 C11.1 | XTAL2.P2 38.47,41.54 37.47,42.55 33.02,42.55 32.2,41.72 C9.1 | J2.5 70.48,15.37 | 70.48,15.37 v70.48,13.97 | J2.3 70.48,15.37 | v68.58,30.48 U6.EP v68.58,29.21 | C19.1 v66.04,26.04 65.09,26.04 C17.1 | C13.1 v66.04,35.56 65.09,35.56 C12.1 | U5.EP v68.58,38.73 | U7.9 v32.38,25.79 | v32.38,25.79 30.55,25.79 C18.2 | U7.8 32.88,26.29 v32.38,25.79 | v81.28,4.45 STATUS.P2
  Top 0.254: U4.90 54.98,38.08 54.98,38.87 54.88,38.97 v54.88,39.5 | U4.5 55.81,52.24 56.26,51.79 C114.2 | 47.79,53.37 U4.25 47.83,53.36 47.83,52.57 48.61,51.79 v50.37,51.79 | C1.2 v12.63,78 12.63,76.85 U1.8 U1.7 10.79,75.56 v10.16,74.93 9.53,74.3 U1.3 | U4.106 57.73,43.12 56.83,42.23 C104.2 | v51.82,48.79 52.21,49.18 U4.14 | U4.78 50.18,38.08 50.18,38.87 49.34,39.71 v49.34,40.01 | U4.45 44.45,47.12 45.59,47.12 46.67,46.04 v46.67,45.09 45.51,43.92 U4.53 | C100.2 58.31,37.15 U4.96 | v41.27,38.73 42.06,39.52 U4.64 | C11.1 C9.1 | C5.1 C6.1 65.08,54.3 v65.41,53.98 | C4.- 20.95,70.41 | U4.116 55.75,47.12 v54.94,47.93 | v30.48,13.34 31.35,13.34 C21.2 32.1,13.34 v33.02,13.34 | U9.1 42.15,14.21 v42.55,14.61 | C20.2 44.82,16.51 v43.81,16.51 | R23.1 v48.26,19.84 | C22.2 46.54,10.79 v45.09,10.79 | R31.1 49.72,10.79 v50.8,10.79 | U4.31 45.41,52.46 45.8,52.07 C115.2 | U4.38 44.44,49.92 v44.83,49.53 | v68.58,68.58 68.8,68.36 C3.2 72.17,68.36 v72.39,68.58 | U2.2 v60.96,72.39 | U6.P2 68.27,30.17 v68.58,30.48 | C10.2 v71.75,39.37 | C17.1 63.82,26.36 v63.5,26.04 63.18,26.36 C16.1 | U5.EP v68.58,40.01 68.27,39.7 U5.P2 | C14.2 v71.75,29.84
  Top 0.406: MICRO_SD.6 v33.6,78.11 | MICRO_SD.P1 v25.4,79.27 | MICRO_SD.P3 v24,70.74 | MICRO_SD.9 v26.31,68.07 | MICRO_SD.P4 v36.96,65.79 | v38.1,78.74 36.92,78.74 MICRO_SD.P2 | USB.5 58.45,14.47 v58.45,14.61 | C4.- 20.95,70.41 | C4.- 20.81,70.41 | 20.95,70.41 21.03,70.48 v22.23,70.48 | C4.- 20.82,70.48 v19.68,70.48 | v22.23,79.38 21.27,79.38 C2.2 20.64,79.38 v19.68,79.38
  Top 0.762: C7.2 27.91,48.29 v27.94,48.26
  Bottom 0.254: C111.2 v44.83,49.53 | C112.2 v51.82,48.79 | C103.2 49.34,40.33 v49.34,40.01 | C108.2 v46.67,45.09 C105.2 | v50.37,51.79 48.94,51.79 C113.2 | v51.82,48.79 C109.2 | v51.82,48.79 51.92,48.9 | C101.2 41.91,38.1 v41.27,38.73 | C102.2 54.88,39.14 v54.88,39.5
  Bottom 0.305: C106.2 54.93,45.4 v54.91,45.41 54.91,46.7 C107.2 v54.94,47.93 C110.2
  other vias: 56.83,41.63 46.67,52.07 56.83,51.79 59.05,37.15 68.58,55.24 78.11,55.24 18.41,39.37 29.21,39.37 13.34,48.26 13.34,53.34 29.21,53.34 33.66,48.26 27.3,57.78 33.66,64.14 33.66,66.04 20.95,66.67 14.61,66.67 9.53,13.97 87,74.3 45.72,76.2 45.72,73.66 45.72,71.12 45.72,68.58 45.72,66.04 45.72,78.74 45.72,63.5 43.18,55.24 48.26,42.55 51.44,45.72 63.5,44.45 74.3,45.72 75.56,23.5 61.59,17.78 20.32,29.84 20.32,19.68 32.38,22.23 54.61,30.48 53.98,22.86 59.05,22.86 59.69,26.04
  pour Route2 (isolate 0.356): 17.14,90.17 5.97,90.17 arc90 0.64,84.84 0.64,5.97 arc90 5.97,0.64 17.14,0.64 arc90 19.68,3.17 19.68,6.99 arc-90 22.23,9.53 73.66,9.53 arc-90 76.2,6.99 76.2,3.17 arc90 78.74,0.64 89.92,0.64 arc90 95.25,5.97 95.25,84.2 arc90 89.92,89.53 78.74,89.53 arc90 76.2,87 76.2,83.19 arc-90 73.66,80.64 22.23,80.64 arc-90 19.68,83.19 19.68,87.63 arc90
  pour Bottom (isolate 0.406): 17.35,90.02 6.17,90.02 arc90 0.84,84.68 0.84,5.82 arc90 6.17,0.48 17.35,0.48 arc90 19.89,3.02 19.89,6.83 arc-90 22.43,9.37 73.86,9.37 arc-90 76.4,6.83 76.4,3.02 arc90 78.94,0.48 90.12,0.48 arc90 95.45,5.82 95.45,84.05 arc90 90.12,89.38 78.94,89.38 arc90 76.4,86.84 76.4,83.03 arc-90 73.86,80.49 22.43,80.49 arc-90 19.89,83.03 19.89,87.48 arc90
  pour Top (isolate 0.406): 17.35,90.02 6.17,90.02 arc90 0.84,84.68 0.84,5.82 arc90 6.17,0.48 17.35,0.48 arc90 19.89,3.02 19.89,6.2 arc-90 23.06,9.37 73.86,9.37 arc-90 76.4,6.83 76.4,3.02 arc90 78.94,0.48 90.12,0.48 arc90 95.45,5.82 95.45,84.05 arc90 90.12,89.38 78.94,89.38 arc90 76.4,86.84 76.4,83.03 arc-90 73.86,80.49 22.43,80.49 arc-90 19.89,83.03 19.89,87.48 arc90
GPIO0  (via drill 0.35)
  Top 0.203: U4.42 42.6,48.32 v41.91,47.62
  Bottom 0.203: JP1.23 9.53,41.27 11.43,41.27 12.06,41.91 12.06,43.81 13.34,45.09 36.2,45.09 36.85,45.74 40.03,45.74 v41.91,47.62
GPIO1  (via drill 0.35)
  Top 0.203: U4.49 37.9,45.52 v37.47,45.09
  Bottom 0.203: JP1.25 9.53,38.73 12.06,38.73 12.7,39.37 12.7,43.18 13.97,44.45 36.83,44.45 v37.47,45.09
GPIO2  (via drill 0.35)
  Top 0.203: U4.50 38.77,45.12 v38.1,44.45
  Bottom 0.203: JP1.27 9.53,36.2 12.7,36.2 13.34,36.83 13.34,42.55 14.61,43.81 37.47,43.81 v38.1,44.45
GPIO3  (via drill 0.35)
  Top 0.203: U4.51 39.64,44.72 v38.73,43.81
  Bottom 0.203: JP1.29 9.53,33.66 13.34,33.66 13.97,34.29 13.97,41.91 15.24,43.18 38.1,43.18 v38.73,43.81
GPIO4  (via drill 0.35)
  Top 0.203: U4.52 40.51,44.32 v39.37,43.18
  Bottom 0.203: JP1.31 9.53,31.11 13.97,31.11 14.61,31.75 14.61,41.27 15.88,42.55 38.73,42.55 v39.37,43.18
GPIO5  (via drill 0.35)
  Top 0.203: U4.55 40.58,43.12 v40.01,42.55
  Bottom 0.203: JP1.33 9.53,28.57 14.61,28.57 15.24,29.21 15.24,40.64 16.51,41.91 39.37,41.91 v40.01,42.55
GPIO6  (via drill 0.35)
  Top 0.203: U4.56 41.45,42.72 v40.64,41.91
  Bottom 0.203: JP1.35 9.53,26.04 15.24,26.04 15.88,26.67 15.88,40.01 17.14,41.27 40.01,41.27 v40.64,41.91
GPIO7  (via drill 0.35)
  Top 0.203: U4.57 42.32,42.32 v41.27,41.27
  Bottom 0.203: JP1.37 9.53,23.5 15.88,23.5 16.51,24.13 16.51,39.37 17.78,40.64 40.64,40.64 v41.27,41.27
GPIO8
  Top 0.203: JP2.23 84.45,41.27 83.82,41.91 83.82,62.23 82.55,63.5 54.61,63.5 53.98,64.14 52.07,64.14 48.21,60.27 U4.24
GPIO9
  Top 0.203: JP2.25 83.82,38.73 83.19,39.37 83.19,61.59 81.92,62.87 53.98,62.87 53.3,63.55 52.12,63.55 48.61,60.04 U4.23
GPIO10
  Top 0.203: JP2.27 83.19,36.2 82.55,36.83 82.55,60.96 81.28,62.23 52.7,62.23 49.41,58.93 U4.21
GPIO11
  Top 0.203: JP2.29 82.55,33.66 81.92,34.29 81.92,60.33 80.64,61.59 52.7,61.59 49.81,58.7 U4.20
GPIO12
  Top 0.203: JP2.31 81.92,31.11 81.28,31.75 81.28,59.69 80.01,60.96 52.7,60.96 50.21,58.46 U4.19
GPIO13
  Top 0.203: JP2.33 81.28,28.57 80.64,29.21 80.64,59.05 79.38,60.33 52.7,60.33 50.61,58.23 U4.18
GPIO14
  Top 0.203: JP2.35 80.64,26.04 80.01,26.67 80.01,58.42 78.74,59.69 52.7,59.69 51.01,57.99 U4.17
GPIO15
  Top 0.203: JP2.37 80.01,23.5 79.38,24.13 79.38,57.78 78.11,59.05 52.7,59.05 51.41,57.76 U4.16
GPIO22  (via drill 0.35)
  Top 0.203: U4.98 59.77,39.92 60.33,39.37 60.33,38.73 v60.96,38.1
  Bottom 0.203: v60.96,38.1 61.59,38.73 61.59,40.01 63.5,41.91 83.19,41.91 83.82,41.27 83.82,40.64 84.45,40.01 87,40.01 JP2.26
GPIO23  (via drill 0.35)
  Top 0.203: U4.99 60.01,40.32 v60.96,39.37
  Bottom 0.203: v60.96,39.37 60.96,40.01 63.5,42.55 87,42.55 JP2.24
I2C0_SCL
  Top 0.203: U1.4 6.35,71.67 6.35,68.58 6.99,67.94
  Top 0.254: JP1.1 6.99,67.94 6.35,67.31 6.35,57.15 6.99,56.52 12.7,56.52 13.97,55.24 20.95,55.24 | U4.48 32.82,45.92 31.11,47.62 31.11,53.98 29.84,55.24 20.95,55.24 | R13.1 20.89,55.18 20.95,55.24
I2C0_SDA
  Top 0.203: U1.5 11.98,72.39 10.79,72.39 9.53,71.12 9.53,61.59 JP1.7
  Top 0.254: JP1.7 9.53,59.05 12.7,59.05 13.34,58.42 13.34,57.15 14.61,55.88 20.95,55.88 | U4.47 33.05,46.32 31.75,47.62 31.75,54.61 30.48,55.88 20.95,55.88 | R12.1 20.95,57.09 20.95,55.88
I2C1_SCL  (via drill 0.35)
  Top 0.254: U4.61 45.64,40.72 v46.35,40.01 | R30.1 91.75,15.88 v91.49,15.88
  Bottom 0.254: v46.35,40.01 48.26,38.1 49.53,36.83 49.53,34.29 46.99,31.75 46.99,22.23 48.26,20.95 58.42,20.95 59.69,19.68 59.69,17.14 60.96,15.88 66.67,15.88 67.94,14.61 67.94,12.7 69.22,11.43 90.17,11.43 91.49,12.75 v91.49,15.88 91.49,34.88 90.17,36.2 JP2.28
I2C1_SDA  (via drill 0.35)
  Top 0.254: U4.60 46.51,41.12 v46.99,40.64 | R29.1 90.17,15.92 v90.76,16.51
  Bottom 0.254: v46.99,40.64 50.16,37.47 50.16,33.66 47.62,31.11 47.62,22.86 48.9,21.59 59.05,21.59 60.33,20.32 60.33,17.78 61.59,16.51 67.31,16.51 68.58,15.24 68.58,13.34 69.85,12.06 89.53,12.06 90.81,13.34 90.81,16.46 v90.76,16.51 90.76,32.43 89.53,33.66 JP2.30
MCU_RESET
  Top 0.203: R15.1 R14.1 C8.2 63.81,45.41 62.9,46.32 U4.114
MOSI
  Top 0.254: U4.27 47.01,55.86 45.09,57.78 42.55,57.78 41.91,58.42 41.91,61.59 41.27,62.23 R10.1
N$1
  Top 0.152: SD_ACTIVITY.A R1.1
N$2
  Top 0.762: C22.1 R31.2 49.51,12.9 USB.SH1 54.05,19.12 54.74,19.81 55.81,19.81 U8.1
  Top 1.016: USB.SH2 60.25,11.05 USB.SH6 USB.SH5 USB.SH4 USB.SH3 54.05,11.05 USB.SH1
N$3
  Top 1.016: JP1.15 JP1.16 18.01,50.16 F1.1
N$4
  Top 0.152: DEBUG2.A R33.1
N$5
  Top 0.152: STATUS.P6 80.51,13 R26.1
  Top 0.203: 80.49,6.95 STATUS.P6
N$6
  Top 0.508: U9.2 U9.4 C21.1 28.13,16.51 J1.2
N$7
  Top 0.152: DEBUG1.A R32.1
N$8
  Top 0.152: R27.1 83.03,11.91 82.55,11.43 81.92,11.43 81.28,10.79 STATUS.P5
N$9
  Top 0.152: R28.1 85.57,11.28 85.09,10.79 82.55,10.79 82.05,10.29 STATUS.P4
N$10  (via drill 0.35)
  Top 0.203: R21.1 41.27,25.4 40.64,24.77 v36.83,24.77 | v35.56,23.5 34.54,24.52 U7.12
  Bottom 0.203: v36.83,24.77 v35.56,23.5
N$11
  Top 0.203: U7.2 39.76,25.79 40.64,26.67 40.64,27.94 41.27,28.57 R19.1
N$12
  Top 0.254: R16.1 74.93,42.39 74.93,41.27 75.25,40.96 C10.1 75.25,37.78 74.93,37.47 74.93,36.35 R17.2
N$13
  Top 0.203: R22.1 38.11,22.23 U7.1
N$14
  Top 0.254: R7.1 59.78,68.9 U2.4
N$15
  Top 0.254: R18.1 74.93,32.87 74.93,31.75 75.25,31.43 C14.1 75.25,28.25 74.93,27.94 74.93,26.82 R20.2
N$16
  Top 0.254: Q1.1 59.3,75.17 58.42,74.3 58.42,71.75 57.47,70.8 R7.2
N$18
  Top 0.254: R3.2 56.59,77.22 Q1.3
RESET
  Top 0.203: J2.10 66.04,13.21 66.04,17.78 66.67,18.41 76.2,18.41 76.83,19.05 76.83,45.72 74.93,47.62 70.86,47.62 R15.2
SCK
  Top 0.254: U4.28 46.61,55.63 45.09,57.15 41.91,57.15 41.27,57.78 41.27,59.05 40.64,59.69 R11.1
SD_ACTIVE_LED  (via drill 0.25, 0.35)
  Top 0.152: U4.122 58.05,49.52 57.15,50.42 53.72,50.42 v53.34,50.8 | R1.2 v17.14,75.56 | v19.05,59.05 30.48,59.05 33.66,55.88 40.01,55.88 42.55,53.34 v43.18,53.34
  Bottom 0.152: v53.34,50.8 53.34,52.07 52.07,53.34 v43.18,53.34 | v19.05,59.05 17.78,59.05 17.14,59.69 v17.14,75.56
SDCD  (via drill 0.3, 0.35)
  Top 0.203: MICRO_SD.10 32.55,64.77 v38.73,64.77 TP8.1 R9.1 | U4.41 41.73,48.72 v41.27,48.26
  Bottom 0.203: v38.73,64.77 41.27,62.23 v41.27,48.26
SDCK  (via drill 0.3, 0.35)
  Top 0.203: TP7.1 30.48,64.77 31.11,64.14 v32.38,64.14
  Top 0.254: v32.49,78.11 32.49,79.27 MICRO_SD.5 | U4.40 38.51,49.12 v37.47,50.16
  Bottom 0.254: v37.47,50.16 37.47,59.05 32.7,63.82 v32.38,64.14 32.49,64.24 32.49,70.48 arc90 32.2,70.77 31.92,70.77 arc-90 31.63,71.06 31.63,75.24 arc-90 31.92,75.52 32.2,75.52 arc90 32.49,75.81 v32.49,78.11
SDCMD  (via drill 0.3, 0.35)
  Top 0.203: v38.73,72.39 TP4.1 R5.1
  Top 0.254: v30.3,78.11 MICRO_SD.3 | U4.33 42.7,51.92 40.64,53.98 36.83,53.98 v36.2,54.61
  Route15 0.203: v38.73,72.39 31.75,72.39 30.3,73.84 v30.3,78.11
  Bottom 0.254: v36.2,54.61 36.2,57.78 30.3,63.68 30.3,70.48 arc-90 30.59,70.77 30.68,70.77 arc90 30.96,71.06 30.96,71.19 arc90 30.68,71.47 30.59,71.47 arc-90 30.3,71.76 30.3,71.89 arc-90 30.59,72.17 30.68,72.17 arc90 30.96,72.46 30.96,72.59 arc90 30.68,72.88 30.59,72.88 arc-90 30.3,73.16 30.3,73.29 arc-90 30.59,73.58 30.68,73.58 arc90 30.96,73.86 30.96,74 arc90 30.68,74.28 30.59,74.28 arc-90 30.3,74.57 30.3,74.7 arc-90 30.59,74.98 30.68,74.98 arc90 30.96,75.27 30.96,75.4 arc90 30.68,75.68 30.59,75.68 arc-90 30.3,75.97 v30.3,78.11
SDDAT0  (via drill 0.3, 0.35)
  Top 0.203: v38.73,74.93 TP3.1 R4.1
  Top 0.254: v34.7,78.11 MICRO_SD.7 | U4.34 41.83,51.52 40.64,52.7 39.32,52.7 v38.73,53.29
  Route15 0.203: v38.73,74.93 35.56,74.93 34.7,75.79 v34.7,78.11
  Bottom 0.254: v34.7,78.11 34.7,75.62 arc-90 34.41,75.34 34.02,75.34 arc90 33.74,75.05 33.74,74.97 arc90 34.02,74.69 34.41,74.69 arc-90 34.7,74.4 34.7,74.32 arc-90 34.41,74.03 34.02,74.03 arc90 33.74,73.75 33.74,73.67 arc90 34.02,73.38 34.41,73.38 arc-90 34.7,73.09 34.7,73.01 arc-90 34.41,72.73 34.02,72.73 arc90 33.74,72.44 33.74,72.36 arc90 34.02,72.08 34.41,72.08 arc-90 34.7,71.79 34.7,71.71 arc-90 34.41,71.42 34.02,71.42 arc90 33.74,71.14 33.74,71.06 arc90 34.02,70.77 34.41,70.77 arc-90 34.7,70.48 34.7,64.36 38.73,60.33 v38.73,53.29
SDDAT1  (via drill 0.35)
  Top 0.203: v38.73,77.47 TP1.1 R2.1
  Top 0.254: v35.79,78.11 MICRO_SD.8 | U4.35 40.91,51.12 v40.01,52.02
  Bottom 0.203: v38.73,77.47 35.79,77.47
  Bottom 0.254: v35.79,78.11 35.79,77.47 35.79,75.67 arc90 36.07,75.39 36.5,75.39 arc-90 36.78,75.1 36.78,75.02 arc-90 36.5,74.73 36.07,74.73 arc90 35.79,74.44 35.79,74.36 arc90 36.07,74.07 36.5,74.07 arc-90 36.78,73.78 36.78,73.7 arc-90 36.5,73.41 36.07,73.41 arc90 35.79,73.12 35.79,73.04 arc90 36.07,72.75 36.5,72.75 arc-90 36.78,72.46 36.78,72.38 arc-90 36.5,72.09 36.07,72.09 arc90 35.79,71.81 35.79,71.72 arc90 36.07,71.43 36.5,71.43 arc-90 36.78,71.14 36.78,71.06 arc-90 36.5,70.77 36.07,70.77 arc90 35.79,70.48 35.79,65.81 40.01,61.59 v40.01,52.02
SDDAT2  (via drill 0.3, 0.35)
  Top 0.203: v38.73,67.31 TP6.1 R8.1
  Top 0.254: U4.36 39.45,50.72 36.83,53.34 34.29,53.34 v33.66,53.98 | v28.09,78.11 MICRO_SD.1
  Route15 0.203: v38.73,67.31 28.73,67.31 v28.09,67.94
  Bottom 0.254: v33.66,53.98 33.66,55.24 28.09,60.81 v28.09,67.94 v28.09,78.11
SDDAT3  (via drill 0.3, 0.35)
  Top 0.203: v38.73,69.85 TP5.1 R6.1
  Top 0.254: v29.21,78.11 v29.2,78.11 MICRO_SD.2 | U4.39 43.53,49.53 39.37,49.53 36.83,52.07 35.51,52.07 v34.92,52.66
  Route15 0.203: v38.73,69.85 30.48,69.85 29.21,71.12 v29.21,78.11
  Bottom 0.254: v29.21,78.11 29.21,62.23 34.92,56.52 v34.92,52.66
SPI1_MISO
  Top 0.203: U4.84 52.61,23.4 51.44,22.23 49.53,22.23 TP16.1 R22.2
SPI1_MOSI
  Top 0.203: U4.82 51.81,28.95 51.44,28.57 TP12.1 R19.2
SPI1_SCK
  Top 0.203: U4.83 52.21,26.17 51.44,25.4 TP14.1 R21.2
SPI_MISO
  Top 0.254: JP1.8 31.11,60.33 33.02,58.42 40.01,58.42 40.64,57.78 40.64,57.15 41.27,56.52 45.09,56.52 46.21,55.39 U4.29
SPI_MOSI
  Top 0.254: R10.2 33.02,62.23 32.38,62.87 JP1.6
SPI_SCK  (via drill 0.35)
  Top 0.254: R11.2 33.66,59.69 31.75,61.59 v13.34,61.59
  Bottom 0.254: JP1.2 11.43,67.94 12.7,66.67 12.7,62.18 13.29,61.59 v13.34,61.59
STAT_B  (via drill 0.25, 0.35)
  Top 0.152: v80.49,16.51 R26.2 | U4.85 53.01,25.1 v53.34,24.77
  Bottom 0.152: v53.34,24.77 54.61,23.5 61.59,23.5 62.87,22.23 62.87,19.68 64.14,18.41 79.38,18.41 80.49,17.3 v80.49,16.51
STAT_G  (via drill 0.25, 0.35)
  Top 0.152: v83.03,16.51 R27.2 | U4.86 53.41,25.97 v53.98,25.4
  Bottom 0.152: v53.98,25.4 55.24,24.13 62.23,24.13 63.5,22.86 63.5,20.32 64.77,19.05 81.92,19.05 83.03,17.93 v83.03,16.51
STAT_R  (via drill 0.25, 0.35)
  Top 0.152: v85.57,16.51 R28.2 | U4.87 53.81,26.84 v54.61,26.04
  Bottom 0.152: v85.57,16.51 85.57,17.93 83.82,19.68 65.41,19.68 64.14,20.95 64.14,23.5 62.87,24.77 55.88,24.77 v54.61,26.04
SWDCLK
  Top 0.203: J2.4 71.12,13.34 71.75,13.97 75.25,13.97 R25.1 77.47,16.19 77.47,46.35 75.5,48.32 U4.119
SWDIO
  Top 0.203: J2.2 72.9,11.43 76.83,11.43 78.13,12.72 78.13,46.97 76.38,48.72 U4.120
SWO
  Top 0.203: J2.6 69.85,10.79 70.48,10.16 76.83,10.16 78.74,12.06 78.74,47.62 77.25,49.12 U4.121
TEMP_SENSE  (via drill 0.35)
  Top 0.203: v45.72,61.27 46.92,61.27 U3.2 | U4.13 52.61,55.34 v52.07,55.88
  Bottom 0.203: v45.72,61.27 46.69,61.27 47.62,60.33 47.62,57.78 48.9,56.52 51.44,56.52 v52.07,55.88
TEMP_SENSE_VDD  (via drill 0.35)
  Top 0.203: U4.30 45.81,54.52 v45.09,55.24 | U3.1 v45.72,59.38
  Bottom 0.203: v45.72,59.38 45.09,58.74 v45.09,55.24
UART0_RX
  Top 0.203: U4.67 45.81,38.95 45.39,39.37 44.78,39.37 44.4,38.99 43.43,38.99 41.91,37.47 13.34,37.47 12.7,38.1 12.7,39.37 12.06,40.01 JP1.24
UART0_TX
  Top 0.203: U4.66 45.41,37.15 45.09,36.83 12.7,36.83 12.06,37.47 JP1.26
UART1_RX
  Top 0.203: U4.70 47.01,35.58 46.35,34.92 JP1.28
UART1_TX
  Top 0.203: U4.71 47.41,35.34 46.35,34.29 13.34,34.29 12.7,33.66 12.7,33.02 12.06,32.38 JP1.30
UART2_RX
  Top 0.203: U4.76 49.41,34.8 48.26,33.66 13.97,33.66 13.34,33.02 13.34,30.48 12.7,29.84 JP1.32
UART2_TX
  Top 0.203: U4.77 49.81,34.57 48.26,33.02 14.61,33.02 13.97,32.38 13.97,27.94 13.34,27.3 JP1.34
UART3_RX  (via drill 0.35)
  Top 0.203: U4.102 61.35,41.52 61.59,41.27 61.59,33.02 v60.96,32.38 | v50.16,32.38 50.14,32.36 15.22,32.36 14.61,31.75 14.61,25.4 13.97,24.77 JP1.36
  Bottom 0.203: v60.96,32.38 v50.16,32.38
UART3_TX  (via drill 0.35)
  Top 0.203: U4.103 61.59,41.92 62.23,41.27 62.23,32.38 v61.59,31.75 | JP1.38 14.61,22.23 15.24,22.86 15.24,31.11 15.83,31.7 v49.53,31.7
  Bottom 0.203: v61.59,31.75 61.55,31.7 v49.53,31.7
USB_N
  Top 0.254: U4.94 56.61,36.67 56.62,36.66 56.62,36.6 56.63,36.58 56.63,18.11 | 56.63,18.11 56.63,14.68 56.5,14.54 USB.2 | U8.2 56.62,18.1 56.63,18.11
USB_P
  Top 0.254: U4.95 57.01,36.67 57.02,36.66 57.02,18.09 | 57.02,18.09 57.02,14.69 57.15,14.55 USB.3 | U8.3 57.8,18.09 57.02,18.09
V_USB  (via drill 0.35)
  Top 0.457: USB.1 55.85,16.48 v55.88,16.51 | U8.4 57.82,19.09 v57.78,19.05 | v45.72,19.05 45.46,19.05 C20.1 45.06,18.81 U9.3
  Bottom 0.457: 55.88,19.05 v57.78,19.05 | v55.88,16.51 55.88,19.05 | 55.88,19.05 51.12,19.05 R24.2 50.48,18.73 50.16,19.05 v45.72,19.05 45.46,19.05 C20.1
  other vias: 50.8,18.73 45.14,18.73
V_USB_SENSE  (via drill 0.2, 0.35)
  Top 0.152: U4.3 56.61,54.75 v56.79,54.94 | R23.2 R24.1 51.76,16.83 52.7,17.78 52.7,19.05 55.88,22.23 55.88,34.29 v54.61,35.56
  Bottom 0.152: v56.79,54.94 55.88,54.02 55.88,38.1 54.61,36.83 v54.61,35.56
VBAT  (via drill 0.35)
  Top 0.254: C3.1 70.38,77.58 | 70.38,77.58 70.27,77.47 64.77,77.47 63.5,76.2 62.44,75.14 61.91,75.14 Q1.2 61.88,71.06 U2.1 U2.5 | v63.5,52.7 62.72,51.92 U4.128 | 70.38,77.58 70.48,77.47 TP2.1 v86.36,77.47
  Bottom 0.254: v63.5,52.7 66.67,49.53 83.82,49.53 84.45,50.16 89.53,50.16 90.81,51.44 90.81,76.2 89.53,77.47 v86.36,77.47
VCC_MCU_3V3  (via drill 0.25, 0.35)
  Top 0.203: U4.97 59.05,39.34 v59.05,38.73 | v50.8,77.47 R2.2 | R4.2 v50.8,74.93 | R5.2 v50.8,72.39 | v50.8,69.85 R6.2 | R8.2 v50.8,67.31 | v50.8,64.77 R9.2 | R14.2 C8.1 63.81,47.3 v63.5,46.99 | J2.1 73.15,16 v73.66,16.51 | C13.2 69.85,35.88 v69.85,37.47 70.08,37.7 U5.P5 | C19.2 69.85,26.36 v69.85,27.94 70.08,28.17 U6.P5 | U7.3 37.72,26.29 v38.1,26.67 C15.1 | U7.7 32.4,26.79 v32.38,26.8 31.56,27.62 C18.1
  Top 0.254: C110.1 56.83,48.66 57.58,47.9 58.86,47.9 U4.118 | v56.83,39.5 56.7,39.37 55.88,39.37 55.41,38.9 U4.91 | C101.1 44.96,38.1 U4.65 | U4.54 44.49,43.52 v44.83,43.18 | U4.79 50.61,39.3 v51.05,39.62 | v44.83,46.33 44.54,46.72 U4.46 | C111.1 45.88,50.32 U4.37 | U4.107 56.82,43.52 C104.1 | U4.32 45.01,52.25 v44.83,52.07 | U2.3 v60.01,72.38 v60.02,72.39 | v55.24,74.93 55.56,75.25 R3.1 57.47,75.25 v57.78,74.93 | C1.1 v10.73,78.04 9.53,76.83 U1.1 | R25.2 75.22,13.02 v74.93,13.31 | v88.9,13.34 89.22,13.02 R29.2 R30.2 93.67,13.02 v93.98,13.34 | R12.2 v24.13,57.15 | R13.2 v24.13,53.98
  Top 0.406: MICRO_SD.4 31.4,80.08 31.09,80.39 27.03,80.39 26.67,80.03 26.67,78.11 25.72,77.16 C2.1 C4.+ | C4.+ 22.09,73.16 v22.23,73.03 | C4.+ 19.82,73.16 v19.68,73.03
  Top 0.61: C2.1 21.27,77.47
  Top 0.762: 25.4,45.52 C7.1
  Top 0.914: C7.1
  Top 1.016: 25.4,45.52 L1.2 21.49,45.74 v19.05,45.74 | C7.1 25.68,45.74 v26.67,45.74 v27.94,45.74
  Bottom 0.254: C102.1 v56.83,39.5 | C108.1 44.83,46.65 v44.83,46.33 | C115.1 v44.83,52.07 | C103.1 50.99,39.69 v51.05,39.62 | C100.1 v59.05,38.73 | C105.1 44.83,43.45 v44.83,43.18
  Bottom 0.406: FB100.1 52.7,44.45 53.34,43.81 53.34,41.91 53.62,41.63 C104.1
  other vias: 56.83,49.25 54.93,41.63 44.13,38.1 46.67,49.53
  pour Route15 (isolate 0.356): 17.14,90.17 5.97,90.17 arc90 0.64,84.84 0.64,5.97 arc90 5.97,0.64 17.14,0.64 arc90 19.68,3.17 19.68,6.99 arc-90 22.23,9.53 73.66,9.53 arc-90 76.2,6.99 76.2,3.17 arc90 78.74,0.64 89.92,0.64 arc90 95.25,5.97 95.25,84.2 arc90 89.92,89.53 78.74,89.53 arc90 76.2,87 76.2,83.19 arc-90 73.66,80.64 22.23,80.64 arc-90 19.68,83.19 19.68,87.63 arc90
VCC_MCU_ANA  (via drill 0.35)
  Top 0.254: U4.6 55.41,52.27 C114.1 54.2,51.79 53.81,52.19 U4.10 | U4.15 51.81,51.81 v51.44,51.44 | U4.26 47.41,51.02
  Top 0.305: 47.41,51.02 v48.9,49.53
  Route15 1.016: C114.1 52.43,51.79 arc90 51.44,50.8 | 51.44,50.8 arc-90 50.16,49.53 v48.9,49.53 | v51.44,51.44 51.44,50.8
  Bottom 0.254: C112.1 51.5,51.44 v51.44,51.44
  Bottom 1.016: FB100.2 C109.1 arc-90 C109.1 48.9,47.62 v48.9,49.53 C113.1
  other vias: 54.93,51.79
VCC_MCU_VDDCORE  (via drill 0.35)
  Top 0.254: U4.115 57.52,46.72 v57.15,46.35
  Bottom 0.254: C107.1 56.83,46.67 v57.15,46.35
  Bottom 0.914: L100.2 57.16,44.5 C106.1 C107.1
VCC_MCU_VSW  (via drill 0.35)
  Top 0.254: L100.1 59.04,47.5 59.03,47.5 58.9,47.5 U4.117
  other vias: 60.6,47.5
XIN0
  Top 0.203: C9.2 36.55,41.27 XTAL2.P3 37.5,40.32 U4.62
XIN32
  Top 0.203: U4.1 58.2,54.19 arc-90 58.57,54.19 59.09,53.67 arc90 59.46,53.67 59.67,53.89 arc90 59.67,54.26 59.16,54.77 arc-90 59.16,55.14 59.28,55.27 XTAL1.P$1 C6.2
  Top 0.254: C6.2
XOUT0
  Top 0.203: U4.63 39.43,39.92 XTAL2.P1 38.16,38.96 37.21,39.9 35.01,39.9 C11.2
XOUT32
  Top 0.203: U4.2 57.06,53.44 57.06,54.2 60.33,57.47 XTAL1.P$2 C5.2

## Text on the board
tPlace: BOARD # / 1 2 3 4
tNames: Samuel Dewan - 2020 | 32.768 kHz | SWD | DEBUG 0 | DEBUG 1 | REV A | BIG-MCU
